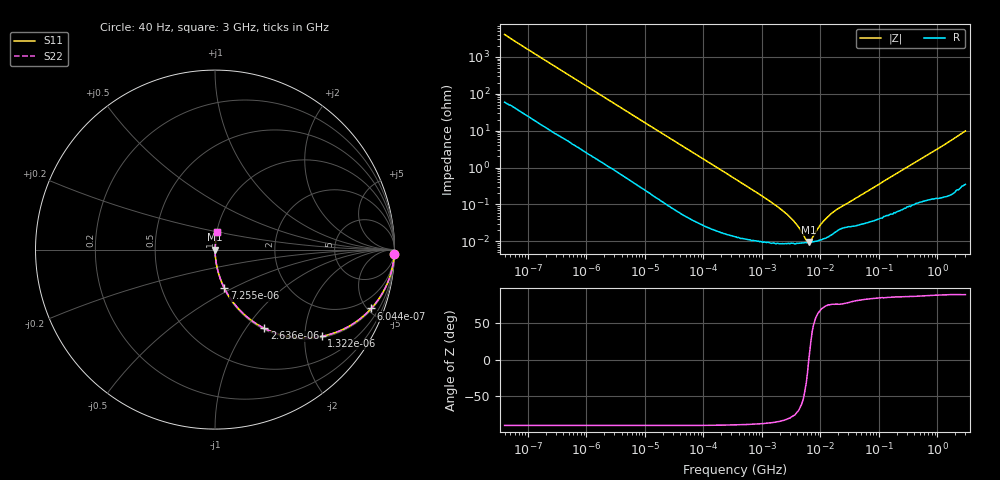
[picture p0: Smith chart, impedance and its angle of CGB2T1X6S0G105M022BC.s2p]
! S-parameter Generated by TDK Corporation
! Copyright(C) 2015 TDK Corporation.
! All Rights Reserved.
! TDK P/N: CGB2T1X6S0G105M022BC (Multilayer Ceramic Chip Capacitors)
! Property: C=1uF
! Size(LxWxT): 1x0.5x0.22mm, 0.039x0.02x0.0087inches
! Model Type: s2p (Touchstone File Format Version 1.0)
! Frequency: DC=Yes Start=0.00004MHz Stop=3000MHz 396points Log-sweep
! Note: This model was converted from impedance.
! Model Generated on Jun. 23, 2015
! Hash(MD5):
! Port Assignments:
!  1 ---| |--- 2
! Applicable Conditions:
!  Temperature = 25 degC
!  DC Bias Voltage = 0 V
!  Small Signal Operation
! Terms and conditions regarding TDK Simulation Models
! (1)This simulation model is being provided solely for informational purposes. Please refer to the specifications of the products in terms of detailed characteristics of such products.
! (2)In no event shall TDK Corporation of any of its subsidiaries be liable for any loss or damage arising, directly or indirectly,
!  From any information contained in this simulation model, including, but not limited to loss or damages arising from any inaccuracies, omissions or errors in connection with such information.
! (3)Any and all copyrights on this simulation model are owned by TDK Corporation.
!  Duplication or redistribution of this simulation model without prior written permission from TDK Corporation is prohibited.
! (4)This simulation model is subject to any modification or change without any prior notice.
! (5)Neither TDK Corporation nor any of its subsidiaries shall make any warranty, express or implied,
!  Including but not limited to the correctness, implied warranties of merchantability and fitness for a particular purpose with respect to this simulation models.
! (6)The use of this simulation model shall be deemed to have consented to the terms and conditions hereof.
# MHz S MA R 50
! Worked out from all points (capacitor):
!   395 points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, 40 Hz to 3 GHz, reference 50 ohm
!   read as one part in series: C = 1 uF near 41.88 Hz
!   lowest |Z| = 9.64 mohm at 6.292 MHz (marker M1)
!   series resonance near 6.326 MHz, so ESL is about 630 pH
!   S11 on the Smith chart (normalised r, x): 40 Hz: 2, -81; 604.4 Hz: 1.08, -5.28; 1.322 kHz: 1.04, -2.42; 2.636 kHz: 1.02, -1.22; 7.255 kHz: 1.01, -0.45; 3 GHz: 1.01, +0.20
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4e-05  0.9993 -1.4  0.0248 87.7  0.0248 87.7  0.9993 -1.4
0.0001912643  0.991 -6.9  0.1196 82.2  0.1196 82.2  0.991 -6.9
0.0006043944  0.9303 -20.6  0.3526 68.5  0.3526 68.5  0.9303 -20.6
0.000834128  0.8807 -27.4  0.46 61.7  0.46 61.7  0.8807 -27.4
0.001321622  0.7655 -39.2  0.6315 49.9  0.6315 49.9  0.7655 -39.2
0.002635842  0.5175 -57.9  0.8476 31.2  0.8476 31.2  0.5175 -57.9
0.004176322  0.3593 -68.1  0.9276 21.1  0.9276 21.1  0.3593 -68.1
0.007255102  0.2185 -76.5  0.9725 12.6  0.9725 12.6  0.2185 -76.5
0.01739424  0.09465 -83.7  0.9941 5.4  0.9941 5.4  0.09465 -83.7
0.05496573  0.03075 -87.4  0.9991 1.8  0.9991 1.8  0.03075 -87.4
0.3464102  0.004971 -88.2  0.9999 0.3  0.9999 0.3  0.004971 -88.2
1.256723  0.001337 -85.8  0.9999 0.1  0.9999 0.1  0.001337 -85.8
2.624455  0.0005586 -81.1  0.9999 0.0  0.9999 0.0  0.0005586 -81.1
3.971241  0.0002808 -71.4  0.9999 0.0  0.9999 0.0  0.0002808 -71.4
5.738865  0.000108 -31.0  0.9999 0.0  0.9999 0.0  0.000108 -31.0
6.292177  9.636e-05 -1.6  0.9999 0.0  0.9999 0.0  9.636e-05 -1.6
7.22376  0.0001222 37.7  0.9999 -0.0  0.9999 -0.0  0.0001222 37.7
9.969551  0.0002802 66.9  0.9999 -0.0  0.9999 -0.0  0.0002802 66.9
15.79611  0.0005892 74.9  0.9998 -0.0  0.9998 -0.0  0.0005892 74.9
150.6385  0.005274 84.0  0.9995 -0.3  0.9995 -0.3  0.005274 84.0
994.0817  0.03159 85.6  0.9981 -1.8  0.9981 -1.8  0.03159 85.6
3000  0.0972 82.4  0.9918 -5.6  0.9918 -5.6  0.0972 82.4
